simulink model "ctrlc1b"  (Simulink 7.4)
settings: Solver=ode15s  StartTime=0.0  StopTime=0.10  MaxStep=1e-4  RelTol=1e-3
libraries: simulink_extras x1

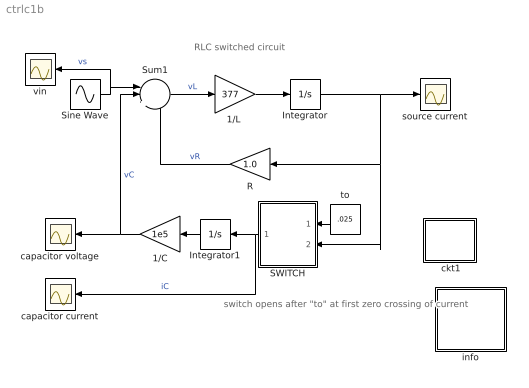
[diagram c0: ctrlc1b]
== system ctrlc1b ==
  note: switch opens after "to" at first zero crossing of current
  note: RLC switched circuit
  " ckt1" : Subsystem
  1/C : Gain  Gain=1e5  ParameterDataType=sfix(16)  ParameterScaling=2^0  OutDataType=sfix(16)  OutScaling=2^0
  "1/L " : Gain  Gain=377  ParameterDataType=sfix(16)  ParameterScaling=2^0  OutDataType=sfix(16)  OutScaling=2^0
  Integrator : Integrator
  Integrator1 : Integrator
  R : Gain  Gain=1.0  ParameterDataType=sfix(16)  ParameterScaling=2^0  OutDataType=sfix(16)  OutScaling=2^0
  SWITCH : Subsystem
  Sine Wave : Sin  Amplitude=120*sqrt(2)  Bias=0  Frequency=2*pi*60  Phase=0  Samples=10  SampleTime=0
  Sum1 : Sum  Inputs=||+--  OutDataType=sfix(16)  OutScaling=2^0
  capacitor current : Scope
  capacitor voltage : Scope
  info : Subsystem
  source current : Scope
  to : Constant  Value=.025  OutDataType=sfix(16)  OutScaling=2^0
  vin : Scope
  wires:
  Sine Wave/1 -> Sum1/1, vin/1  "vs"
  R/1 -> Sum1/3  "vR"
  1/C/1 -> Sum1/2, capacitor voltage/1  "vC"
  SWITCH/1(iC) -> Integrator1/1, capacitor current/1  "iC"
  Integrator1/1 -> 1/C/1
  to/1 -> SWITCH/1(to)
  Sum1/1 -> "1/L "/1  "vL"
  "1/L "/1 -> Integrator/1
  Integrator/1 -> source current/1, SWITCH/2(I), R/1  "i"

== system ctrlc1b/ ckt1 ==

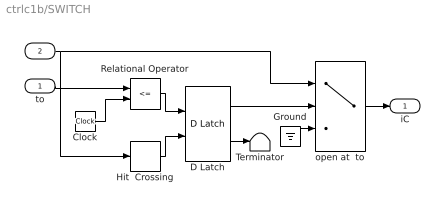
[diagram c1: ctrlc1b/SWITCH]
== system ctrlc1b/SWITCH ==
  to : Inport  OutDataType=sfix(16)  OutScaling=2^0
  I : Inport  Port=2  OutDataType=sfix(16)  OutScaling=2^0
  Clock : Clock
  D Latch : simulink_extras/Flip Flops/D Latch  SystemSampleTime=-1
  Ground : Ground
  Hit  Crossing : HitCross
  Relational Operator : RelationalOperator  Operator=<=
  Terminator : Terminator
  open at  to : Switch  Threshold=0.5
  iC : Outport
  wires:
  Hit  Crossing/1 -> D Latch/2
  Relational Operator/1 -> D Latch/1
  Clock/1 -> Relational Operator/2
  to/1 -> Relational Operator/1
  D Latch/2 -> Terminator/1
  Ground/1 -> open at  to/3
  D Latch/1 -> open at  to/2
  open at  to/1 -> iC/1
  I/1 -> open at  to/1, Hit  Crossing/1

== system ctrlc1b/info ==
  note: RLC switched circuit
  note: A series RL circuit operates under sinusoidal voltage excitation for a specified length of time "to" when, at the first subsequent current zero, a circuit breaker suddenly opens inserting a capacitance C in series with the RL circuit. The circuit breaker is simulated by means of a switch block activated by a D latch flipflop block which determines a zero-hit crossing immediately following the commanded time "to". The source current i as well as the capacitor current iC and voltage vC are exhibited as functions of time.
